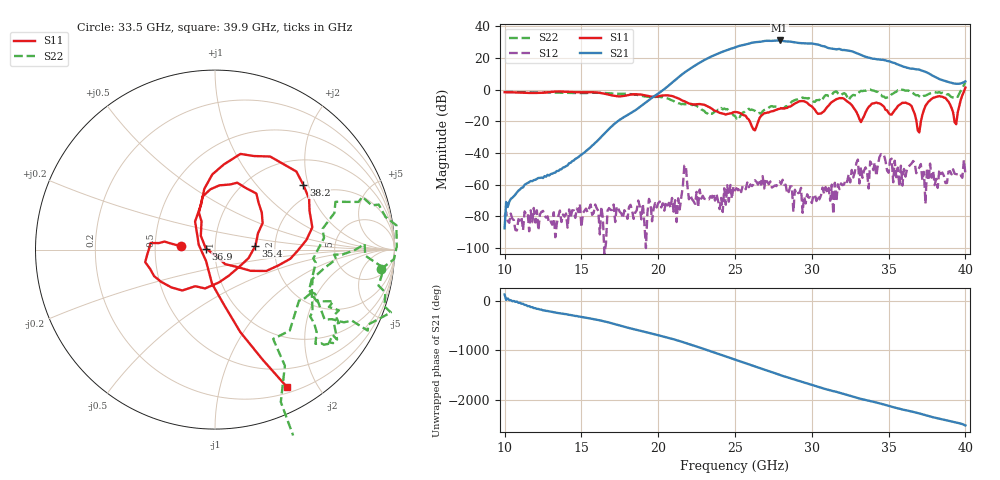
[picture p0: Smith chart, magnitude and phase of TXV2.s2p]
!Keysight Technologies,M9808A,MY58100618,A.14.70.03
!Date: Monday, February 27, 2023 13:18:48
!Correction: S11(C  2-Port  )
!S21(C  2-Port  )
!S12(C  2-Port  )
!S22(C  2-Port  )
!S2P File: Measurements: S11, S21, S12, S22:
# Hz S  RI  R 50
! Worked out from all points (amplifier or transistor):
!   301 points, 10 GHz to 40 GHz, reference 50 ohm
!   highest |S21| = 31.1 dB at 27.9 GHz (marker M1)
!   |S21| within 3 dB of that: 25.49 GHz to 30.53 GHz (5.044 GHz wide, 18 % of centre)
!   unconditionally stable (mu >= 1): start of sweep to 33.56 GHz; 33.94 GHz to 35.74 GHz; 36.01 GHz to 39.74 GHz
!   at 15 GHz: K = 150071.47, MAG = -31.9 dB, |S12| = -86.9 dB
!   at 25 GHz: K = 32.74, MAG = 27.0 dB, |S12| = -63.6 dB
!   at 40 GHz: K = 91.30, MSG = 29.1 dB, |S12| = -52.9 dB
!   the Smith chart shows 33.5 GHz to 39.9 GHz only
!   S11 on the Smith chart (normalised r, x): 33.5 GHz: 0.68, +0.03; 35.4 GHz: 1.58, +0.07; 36.9 GHz: 0.90, +0.01; 38.2 GHz: 1.62, +1.86; 39.9 GHz: 0.27, -1.62
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1e10  0.6984 0.4647  -2.4e-05 3.42e-05  -9.32e-05 -3.84e-05  0.08 0.8435
1.5e10  0.6645 -0.4945  0.00749 0.00469  3.96e-05 2.16e-05  0.7711 0.156
2e10  -0.1652 -0.5983  0.6967 0.2993  -4.15e-06 0.000259  0.2076 -0.5544
2.34e10  -0.2494 -0.1003  5.205 9.566  0.000334 0.000273  -0.0921 -0.1489
2.42e10  -0.1749 0.0238  14.68 -6.187  0.000115 -7.36e-05  -0.1867 -0.1496
2.5e10  -0.1366 0.1453  -6.207 -20.79  7.74e-05 0.000656  -0.134 -0.0639
2.58e10  -0.0961 0.0788  -27.24 5.454  0.000847 0.000822  -0.206 0.09
2.66e10  0.1239 -0.0338  4.471 32.37  0.00119 0.000855  -0.1191 0.1425
2.73e10  0.1913 -0.0663  34.65 4.624  0.00122 0.000354  -0.0677 0.2867
2.79e10  0.1966 -0.1539  20.56 -29.64  0.00111 0.00061  0.0112 0.2716
2.89e10  0.0644 -0.3618  -28.54 -13.87  0.000683 -0.000114  0.2384 0.4074
3e10  0.1166 -0.2748  -6.645 28.08  2.08e-05 0.000263  0.203 0.4179
3.08e10  -0.147 -0.1505  21.27 10.24  0.00048 0.000187  0.5751 0.1578
3.18e10  -0.2674 -0.4731  10.81 -16.21  -0.000548 0.000468  0.5255 0.4976
3.27e10  0.023 -0.2799  -11.74 -10.6  -0.00146 0.000847  0.6857 -0.0371
3.35e10  -0.1917 0.0194  -10.09 4.312  -0.00117 0.00332  0.9225 -0.1096
3.5e10  0.0226 -0.1827  6.262 4.985  -0.000752 -0.00225  0.5228 -0.2298
3.54e10  0.2256 0.0218  6.927 0.4926  -0.00502 0.00275  0.7177 -0.4053
3.69e10  -0.051 0.00602  -1.252 -4.218  0.000479 -0.00272  0.6749 -0.054
3.82e10  0.492 0.3611  -1.909 1.281  0.000786 -8.41e-05  0.6558 -0.4759
3.99e10  0.4001 -0.7649  1.653 0.5025  0.00585 0.00126  0.4852 -1.308
4e10  0.587 -1.015  1.837 0.078  -0.00181 0.00138  0.6814 -1.604
